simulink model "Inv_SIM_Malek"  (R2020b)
settings: Solver=FixedStepDiscrete  StartTime=0.0  StopTime=0.06  FixedStep=4e-6  RelTol=1e-4
undefined symbols (not defined in the file): bridge, D1, Delta, phase, pulses, Three
libraries: powerlib x24, dspstat3 x1, powerlib_meascontrol x1

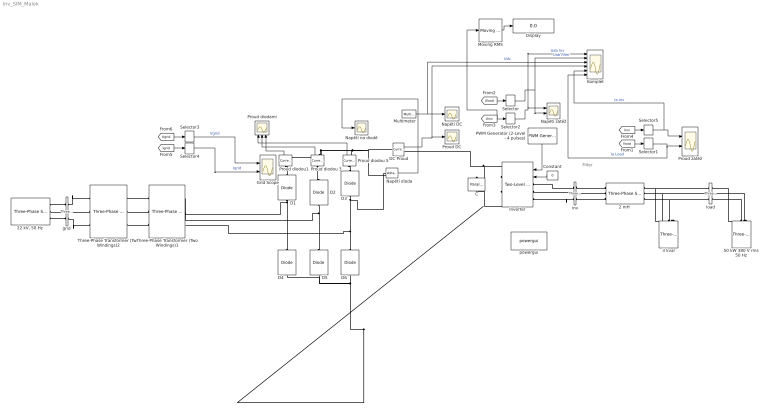
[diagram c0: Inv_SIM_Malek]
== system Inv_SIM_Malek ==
  note: Filter
  "2 mH " : powerlib/Elements/Three-Phase Series RLC Branch  LConnTagsString=A|B|C  RConnTagsString=A|B|C  BranchType=L  Resistance=0  Inductance=2e-3  Capacitance=inf  Measurements=None
  "22 kV, 50 Hz " : powerlib/Electrical Sources/Three-Phase Source  InternalConnection=Yg  VoltagePhases=off  Voltage=22e3  PhaseAngle=0  Voltage_phases=[25e3 25e3 25e3]/sqrt(3)  PhaseAngles_phases=[0 -120 +120]  Frequency=50  NonIdealSource=on  SpecifyImpedance=on  Resistance=25e3^2/10e6/5  Inductance=25e3^2/10e6/377  ShortCircuitLevel=10e6  BaseVoltage=25e3  XRratio=5  BusType=swing  Pref=0  Qref=0  Prefabc=[10e3, 10e3, 10e3]  Qrefabc=[0, 0, 0]  Qmin=-inf  Qmax=inf
  3 kvar : powerlib/Elements/Three-Phase Series RLC Load  LConnTagsString=A|B|C  Configuration=Delta  NominalVoltage=690  Vabc=[1e3 1e3 1e3]  Vabcp=[1e3 1e3 1e3]  NominalFrequency=50  UnbalancedPower=off  ActivePower=0  InductivePower=0  CapacitivePower=3e3  Pabc=[10e3 9e3 11e3]  QLabc=[100 90 110]  QCabc=[100 90 110]  Pabcp=[10e3 9e3 11e3]  QLabcp=[100 90 110]  QCabcp=[100 90 110]  Measurements=None  LoadType=constant Z
  50 kW 380 V rms 50 Hz : powerlib/Elements/Three-Phase Parallel RLC Load  LConnTagsString=A|B|C  Configuration=Delta  NominalVoltage=380  Vabc=[1e3 1e3 1e3]  Vabcp=[1e3 1e3 1e3]  NominalFrequency=50  UnbalancedPower=off  ActivePower=150e3  InductivePower=0  CapacitivePower=0  Pabc=[10e3 9e3 11e3]  QLabc=[100 90 110]  QCabc=[100 90 110]  Pabcp=[10e3 9e3 11e3]  QLabcp=[100 90 110]  QCabcp=[100 90 110]  Measurements=None  LoadType=constant Z
  C : powerlib/Elements/Parallel RLC Branch  LConnTagsString=a  RConnTagsString=__new0  BranchType=C  Resistance=inf  Inductance=inf  SetiL0=off  InitialCurrent=0  Capacitance=5000e-06  Setx0=on  InitialVoltage=800  Measurements=Branch voltage
  Constant : Constant  Value=0
  D{1..6} (6 alike) : powerlib/Power Electronics/Diode  Ron=0.026e-3  Lon=0  Vf=1.8  IC=0  UseSnubber=0  Rs=0.005  Cs=1*0.047e-6  Measurements=off
  DC Proud : powerlib/Measurements/Current Measurement  PhasorSimulation=off  OutputType=Complex  PSBequivalent=0
  Display : Display
  Grid Scope : Scope  NumInputPorts=2
  Inverter : powerlib/Power Electronics/Two-Level Converter  ModelType=Switching devices  Ron=1e-3  Rs=1e6  Cs=inf  Vforward=[0,0]  Ron_Diode=1e-3  Rs_Diode=1e6  Cs_Diode=inf  Vf_Diode=1e-3  Rs_CurrentSource=inf
  Komplet : Scope  NumInputPorts=6
  Moving RMS : dspstat3/Moving RMS  Method=Sliding window  ForgettingFactorPort=off  SpecifyWindowLength=on  WindowLength=4  ForgettingFactor=0.9  SimulateUsing=Code generation
  Multimeter : powerlib/Measurements/Multimeter  PhasorSimulation=off  OutputType=Complex  sel=1  L=1  Gain=1  yselected={'Ub: C'};  PSBOutputType=1  PSBequivalent=0  AxesSetting=[0,0.1,-100,100]  Display=0  SavedBlockNames=-11
  Napětí DC : Scope
  Napětí dioda : powerlib/Measurements/Voltage Measurement  PhasorSimulation=off  OutputType=Complex  PSBequivalent=0
  Napětí na diodě : Scope
  Napětí zátěž : Scope  NumInputPorts=2
  PWM Generator (2-Level - 4 pulses) : powerlib_meascontrol/Pulse & Signal Generators/PWM Generator (2-Level)  ModulatorType=Three-phase bridge (6 pulses)  ModulatorMode=Unsynchronized  Fc=2000  Pc=90  nF=27  MinMax="[ -1  1 ]"  SamplingTechnique=Natural  ModulatingSignals=on  m=0.8  Freq=50  Phase=0  Ts=4e-6  ShowCarrierOutport=off
  Proud DC : Scope
  Proud diodami : Scope  NumInputPorts=3
  Proud diodou 3 : powerlib/Measurements/Current Measurement  PhasorSimulation=off  OutputType=Complex  PSBequivalent=0
  Proud diodou 5 : powerlib/Measurements/Current Measurement  PhasorSimulation=off  OutputType=Complex  PSBequivalent=0
  Proud diodou1 : powerlib/Measurements/Current Measurement  PhasorSimulation=off  OutputType=Complex  PSBequivalent=0
  Proud zátěž : Scope  NumInputPorts=2
  Selector : Selector  IndexMode=Zero-based  InputPortWidth=3  IndexOptions=Index vector (dialog)  Indices=0  OutputSizes=1
  Selector1 : Selector  IndexMode=Zero-based  InputPortWidth=3  IndexOptions=Index vector (dialog)  Indices=1  OutputSizes=1
  Selector2 : Selector  IndexMode=Zero-based  InputPortWidth=3  IndexOptions=Index vector (dialog)  Indices=2  OutputSizes=1
  Selector3 : Selector  IndexMode=Zero-based  InputPortWidth=3  IndexOptions=Index vector (dialog)  Indices=0  OutputSizes=1
  Selector4 : Selector  IndexMode=Zero-based  InputPortWidth=3  IndexOptions=Index vector (dialog)  Indices=0  OutputSizes=1
  Selector5 : Selector  IndexMode=Zero-based  InputPortWidth=3  IndexOptions=Index vector (dialog)  Indices=1  OutputSizes=1
  Three-Phase Transformer (Two Windings)1 : powerlib/Elements/Three-Phase Transformer (Two Windings)  Winding1Connection=Delta (D1)  Winding2Connection=Yg  CoreType=Three single-phase transformers  SetSaturation=off  Hysteresis=off  DataFile='hysteresis'  SetInitialFlux=off  Measurements=None  UNITS=pu  NominalPower=[ 150e3 , 50 ]  Winding1=[ 400 , 0.002 , 0.08 ]  Winding2=[ 666 , 0.002 , 0.08 ]  Rm=500  Lm=500  L0=0.5  Saturation=[ 0,0 ; 0.0024,1.2 ; 1.0,1.52 ]  InitialFluxes=[ 0.8 , -0.8 , 0.7 ]  BreakLoop=off  DiscreteSolver=Trapezoidal iterative  DataType=off  TransfoNumber=1
  Three-Phase Transformer (Two Windings)2 : powerlib/Elements/Three-Phase Transformer (Two Windings)  Winding1Connection=Delta (D1)  Winding2Connection=Yg  CoreType=Three single-phase transformers  SetSaturation=off  Hysteresis=off  DataFile='hysteresis'  SetInitialFlux=off  Measurements=None  UNITS=pu  NominalPower=[ 630e3 , 50 ]  Winding1=[ 22e3 , 0.002 , 0.08 ]  Winding2=[ 400 , 0.002 , 0.08 ]  Rm=500  Lm=500  L0=0.5  Saturation=[ 0,0 ; 0.0024,1.2 ; 1.0,1.52 ]  InitialFluxes=[ 0.8 , -0.8 , 0.7 ]  BreakLoop=off  DiscreteSolver=Trapezoidal iterative  DataType=off  TransfoNumber=1
  grid : powerlib/Measurements/Three-Phase V-I Measurement  VoltageMeasurement=phase-to-ground  SetLabelV=on  LabelV=Vgrid  Vpu=off  VpuLL=off  CurrentMeasurement=yes  SetLabelI=on  LabelI=Igrid  Ipu=off  Pbase=1e3  Vbase=380  OutputType=Magnitude  PhasorSimulation=off  PSBequivalent=0
  inv : powerlib/Measurements/Three-Phase V-I Measurement  VoltageMeasurement=phase-to-phase  SetLabelV=on  LabelV=Uinv  Vpu=off  VpuLL=off  CurrentMeasurement=yes  SetLabelI=on  LabelI=Iinv  Ipu=off  Pbase=1e3  Vbase=380  OutputType=Magnitude  PhasorSimulation=off  PSBequivalent=0
  load : powerlib/Measurements/Three-Phase V-I Measurement  VoltageMeasurement=phase-to-phase  SetLabelV=on  LabelV=Uload  Vpu=off  VpuLL=off  CurrentMeasurement=yes  SetLabelI=on  LabelI=Iload  Ipu=off  Pbase=1e3  Vbase=380  OutputType=Magnitude  PhasorSimulation=off  PSBequivalent=0
  powergui : powerlib/powergui  Priority=1  SimulationMode=Discrete  SampleTime=4e-6  frequency=60  Iterations=50  frequencyindice=50  Pbase=100e6  ErrMax=1e-4  UnitsV=kV  UnitsW=MW  buscounter=0  FunctionMessages=off  echomessages=off  EnableUseOfTLC=off  CurrentSourceSwitches=off  DisableSnubberDevices=off  DisableRonSwitches=off  DisableVfSwitches=off  DisplayEquations=off  AutomaticDiscreteSolvers=off  SolverType=Tustin/Backward Euler (TBE)  Interpol=off  ExternalGateDelay=off  methode=off  Ts=100  x0status=blocks  SPID=off  SwTol=0  HookPort=off  NonlinearTolerance=1e-4  nMaxIteration=100  ContinueOnMaxIteration=off  RestoreLinks=warning  ResistiveCurrentMeasurement=off  Frange=[0:2:500]  Ylog=off  Xlog=on  ShowGrid=off  save=off  variable=ZData  structure=0  ZoomFFT=off  StartTime=0.0  cycles=1  DisplayStyle=1  fundamental=60  FreqAxis=off  MaxFrequency=1000  frequencyindicesteady=1  RmsSteady=1  display=off
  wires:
  [Uload] -> Selector/1
  [Uinv] -> Moving RMS/1, Selector2/1
  [Iload] -> Selector1/1
  Constant/1 -> Inverter/2
  Selector/1 -> Napětí zátěž/2, Komplet/2  "Uab filter"
  Selector1/1 -> Komplet/6, Proud zátěž/2  "Ia Load"
  Selector2/1 -> Komplet/1, Napětí zátěž/1  "Uab Inv"
  [Ugrid] -> Selector3/1
  [Igrid] -> Selector4/1
  Selector3/1 -> Grid Scope/1  "Vgrid"
  Selector4/1 -> Grid Scope/2  "Igrid"
  PWM Generator (2-Level - 4 pulses)/1 -> Inverter/1
  Multimeter/1 -> Komplet/3, Napětí DC/1  "Udc"
  DC Proud/1 -> Komplet/4, Proud DC/1
  [Iinv] -> Selector5/1
  Selector5/1 -> Komplet/5, Proud zátěž/1  "Ia Inv"
  Napětí dioda/1 -> Napětí na diodě/1
  Proud diodou 5/1 -> Proud diodami/1
  Moving RMS/1 -> Display/1
  Proud diodou 3/1 -> Proud diodami/2
  Proud diodou1/1 -> Proud diodami/3
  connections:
  50 kW 380 V rms 50 Hz/LConn2 -- load/RConn2
  load/RConn1 -- 50 kW 380 V rms 50 Hz/LConn1
  load/RConn3 -- 50 kW 380 V rms 50 Hz/LConn3
  "2 mH "/RConn3 -- 3 kvar/LConn3 -- load/LConn3
  "2 mH "/RConn2 -- 3 kvar/LConn2 -- load/LConn2
  "2 mH "/RConn1 -- 3 kvar/LConn1 -- load/LConn1
  Inverter/LConn1 -- inv/LConn1
  inv/LConn2 -- Inverter/LConn2
  inv/LConn3 -- Inverter/LConn3
  Inverter/RConn2 -- D4/LConn1 -- D5/LConn1 -- D6/LConn1 -- C/RConn1
  inv/RConn1 -- "2 mH "/LConn1
  inv/RConn2 -- "2 mH "/LConn2
  inv/RConn3 -- "2 mH "/LConn3
  grid/LConn1 -- "22 kV, 50 Hz "/RConn1
  "22 kV, 50 Hz "/RConn2 -- grid/LConn2
  "22 kV, 50 Hz "/RConn3 -- grid/LConn3
  grid/RConn1 -- Three-Phase Transformer (Two Windings)2/LConn1
  Three-Phase Transformer (Two Windings)2/LConn2 -- grid/RConn2
  grid/RConn3 -- Three-Phase Transformer (Two Windings)2/LConn3
  Three-Phase Transformer (Two Windings)2/RConn1 -- Three-Phase Transformer (Two Windings)1/LConn1
  Three-Phase Transformer (Two Windings)1/LConn2 -- Three-Phase Transformer (Two Windings)2/RConn2
  Three-Phase Transformer (Two Windings)2/RConn3 -- Three-Phase Transformer (Two Windings)1/LConn3
  D3/LConn1 -- Three-Phase Transformer (Two Windings)1/RConn3 -- D6/RConn1 -- Napětí dioda/LConn1
  Proud diodou 5/RConn1 -- Napětí dioda/LConn2 -- DC Proud/LConn1 -- Proud diodou1/RConn1 -- Proud diodou 3/RConn1
  D2/LConn1 -- Three-Phase Transformer (Two Windings)1/RConn2 -- D5/RConn1
  D1/LConn1 -- Three-Phase Transformer (Two Windings)1/RConn1 -- D4/RConn1
  Inverter/RConn1 -- DC Proud/RConn1 -- C/LConn1
  D3/RConn1 -- Proud diodou 5/LConn1
  Proud diodou 3/LConn1 -- D2/RConn1
  D1/RConn1 -- Proud diodou1/LConn1
